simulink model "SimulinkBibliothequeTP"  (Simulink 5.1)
settings: Solver=ode45  StartTime=0.0  StopTime=T  FixedStep=0.1  MaxStep=0.1  MinStep=0.01  RelTol=0.1  AbsTol=0.01
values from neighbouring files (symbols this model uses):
  theta1 = theta1_last+n*Deltatheta1    [GestionGUI.m]    (also in ModeleGeometriqueDirect.m = Theta(1); ModeleGeometriqueInverse.m = alpha - beta; SimulationRobotSCARA.m = 1.57079632679)
  theta2 = theta2_last+n*Deltatheta2    [GestionGUI.m]    (also in ModeleGeometriqueDirect.m = Theta(2); ModeleGeometriqueInverse.m = acos((x^2+y^2-l1^2-l2^2)/(2*l1*l2)); SimulationRobotSCARA.m = 1.57079632679)
undefined symbols (not defined in the file or in its folder): Ki2, Kp2
libraries: simulink x1

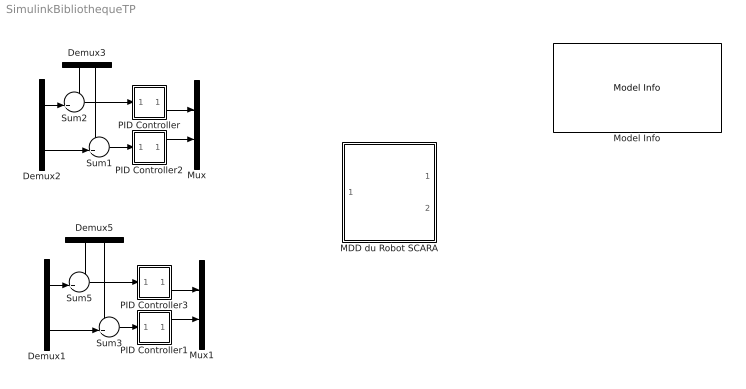
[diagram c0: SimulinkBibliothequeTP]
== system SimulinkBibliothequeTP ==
  Demux1 : Demux  Outputs=2
  Demux2 : Demux  Outputs=2
  Demux3 : Demux  Orientation=down  Outputs=2
  Demux5 : Demux  Orientation=down  Outputs=2
  MDD du Robot SCARA : Subsystem  Tag=Robot  Description=Robot
  Model Info : simulink/Model-Wide Utilities/Model Info  InitialBlockCM=None  BlockCM=None  Frame=on  DisplayStringWithTags="Blocs Simulink que vous pouvez  directement utiliser dans votre TP."  HorizontalTextAlignment=Left  LeftAlignmentValue=0.02  SourceBlockDiagram=SimulinkBibliothequeTP  TagMaxNumber=20
  Mux : Mux  Inputs=[1 1]
  Mux1 : Mux  Inputs=[1 1]
  PID Controller : Subsystem  AncestorBlock=simulink_extras/Additional Linear/PID Controller  mask(PID Controller){P=1, I=1}
      mask prompts: P "Proportional:"; I "Integral:"
      mask help: Enter expressions for proportional, integral P+I/s
  PID Controller1 : Subsystem  AncestorBlock=simulink_extras/Additional Linear/PID Controller  mask(D Controller){D=1}
      mask prompts: D "Derivative:"
      mask help: Enter expression derivative term. Ds
  PID Controller2 : Subsystem  AncestorBlock=simulink_extras/Additional Linear/PID Controller  mask(PID Controller){P=Kp2, I=Ki2}
      mask prompts: P "Proportional:"; I "Integral:"
      mask help: Enter expressions for proportional, integral P+I/s
  PID Controller3 : Subsystem  AncestorBlock=simulink_extras/Additional Linear/PID Controller  mask(D Controller){D=1}
      mask prompts: D "Derivative:"
      mask help: Enter expression derivative term. Ds
  Sum{1..3,5} (4 alike) : Sum  Inputs=-+|
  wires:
  PID Controller/1(Out_1) -> Mux/1
  Sum2/1 -> PID Controller/1(In_1)
  Demux3/1 -> Sum2/1
  Demux3/2 -> Sum1/1
  Demux2/1 -> Sum2/2
  Demux2/2 -> Sum1/2
  ? -> Demux2/1
  Sum1/1 -> PID Controller2/1(In_1)
  PID Controller2/1(Out_1) -> Mux/2
  Mux/1 -> ?
  ? -> Demux1/1
  PID Controller3/1(Out_1) -> Mux1/1
  Sum5/1 -> PID Controller3/1(In_1)
  Demux5/1 -> Sum5/1
  Demux5/2 -> Sum3/1
  Demux1/1 -> Sum5/2
  Demux1/2 -> Sum3/2
  Sum3/1 -> PID Controller1/1(In_1)
  PID Controller1/1(Out_1) -> Mux1/2
  ? -> Demux5/1
  Mux1/1 -> ?
  ? -> Demux3/1

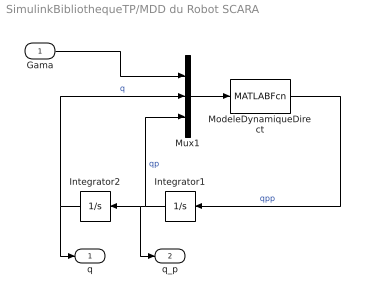
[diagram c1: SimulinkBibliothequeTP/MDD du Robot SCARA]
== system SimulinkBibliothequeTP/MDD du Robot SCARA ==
  Gama : Inport
  Integrator1 : Integrator  Orientation=left  InitialCondition=zeros(1,2)
  Integrator2 : Integrator  Orientation=left  InitialCondition=[theta1, theta2]
  ModeleDynamiqueDirect : MATLABFcn  MATLABFcn=ModeleDynamiqueDirect  OutputDimensions=2
  Mux1 : Mux  Inputs=[2 2 2]
  q : Outport
  q_p : Outport  Port=2
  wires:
  Mux1/1 -> ModeleDynamiqueDirect/1
  Integrator1/1 -> Mux1/3, Integrator2/1, q_p/1  "qp"
  ModeleDynamiqueDirect/1 -> Integrator1/1  "qpp"
  Integrator2/1 -> Mux1/2, q/1  "q"
  Gama/1 -> Mux1/1

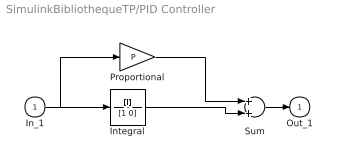
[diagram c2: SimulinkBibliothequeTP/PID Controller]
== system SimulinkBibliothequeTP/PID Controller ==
  In_1 : Inport
  Integral : TransferFcn  Numerator=[I]  Denominator=[1 0]
  Proportional : Gain  Gain=P
  Sum : Sum
  Out_1 : Outport  InitialOutput=0
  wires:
  Proportional/1 -> Sum/1
  Integral/1 -> Sum/2
  In_1/1 -> Integral/1, Proportional/1
  Sum/1 -> Out_1/1

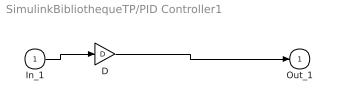
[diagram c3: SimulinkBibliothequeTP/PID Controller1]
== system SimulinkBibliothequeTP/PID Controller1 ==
  In_1 : Inport
  D : Gain  Gain=D
  Out_1 : Outport  InitialOutput=0
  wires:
  In_1/1 -> D/1
  D/1 -> Out_1/1

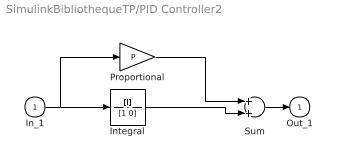
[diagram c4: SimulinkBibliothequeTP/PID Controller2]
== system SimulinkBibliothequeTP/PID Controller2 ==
  In_1 : Inport
  Integral : TransferFcn  Numerator=[I]  Denominator=[1 0]
  Proportional : Gain  Gain=P
  Sum : Sum
  Out_1 : Outport  InitialOutput=0
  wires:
  Proportional/1 -> Sum/1
  Integral/1 -> Sum/2
  In_1/1 -> Integral/1, Proportional/1
  Sum/1 -> Out_1/1

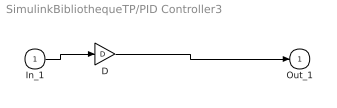
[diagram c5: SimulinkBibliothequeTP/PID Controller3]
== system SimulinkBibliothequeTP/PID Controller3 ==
  In_1 : Inport
  D : Gain  Gain=D
  Out_1 : Outport  InitialOutput=0
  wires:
  In_1/1 -> D/1
  D/1 -> Out_1/1
